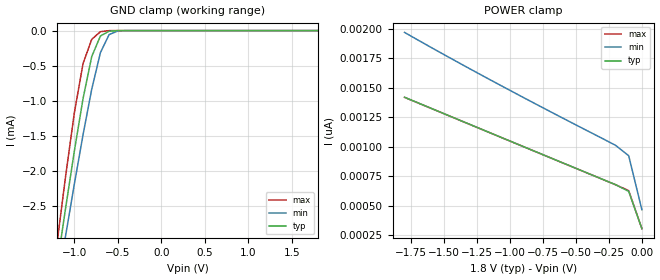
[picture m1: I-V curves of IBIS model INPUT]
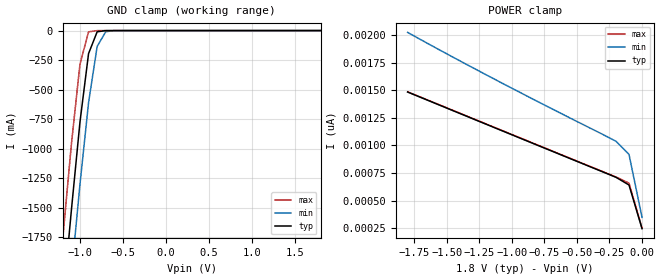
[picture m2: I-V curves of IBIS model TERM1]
|   PERICOM SEMICONDUCTOR CORP
|   IBIS Model of PI3CH360
|   Product Family: 3CH
|   TSSOP (L) Package
[IBIS Ver] 3.2
[Comment char] |_char
[File Name] pi3ch360_l_18v.ibs
[File Rev] 1.0
[Source] File originated at Pericom Semiconductor Corp.
[Date] 3/18/15
[Disclaimer] (C) Copyright PERICOM Semiconductor Corporation
   All rights reserved
  Pericom Semiconductor Corporation hereby grants the user of
  this IBIS model a non-exclusive, nontransferable license to
  use this IBIS model under the following terms.
  This IBIS model is provided on an "AS IS" basis and Pericom
  makes absolutely no warranty with respect to the information
  contained herein. PERICOM DISCLAIMS AND CUSTOMER WAIVES ALL
  WARRANTIES, EXPRESSED OR IMPLIED, INCLUDING WARRANTIES OF
  MERCHANTABILITY OR FITNESS FOR A PARTICULAR PURPOSE. The
  entire risk as to quality and performance is with the customer.
  Accordingly, in no event shall the company be liable for any
  damages, whether in contract or tort, including any lost
  profits or other incidental, consequential, exemplary, or
  punitive damages arising out of the use or application of the
  IBIS model provided in this package. Further, Pericom reserves
  the right to make changes without notice to any product herein
  to improve reliability, function, or design. Pericom does not
  convey any license under patent rights or any other intellectual
  property rights, including those of third parties.
  The user is granted this license only to use the IBIS model
  and is not granted rights to sell, load, rent, lease or license
  the IBIS model in whole or in part, or in modified form to anyone
  other than user. User may modify the IBIS model to suit its specific
  application but rights to derivative works and such modifications
  shall belong to Pericom.
  Pericom is not obligated to provide maintenance or support
  for the licensed IBIS model.
  Contact Pericom at ATTN: APPLICATION ENGINEERING / IBIS MODELS
  3545 North First Street, San Jose, CA 95134
[Component] PI3CH360
[Manufacturer] Pericom Semiconductor Corp.
[Package]
| variable   typ   min   max
R_pkg   0.05666ohm   0.05334ohm   0.05997ohm
L_pkg   2.99150nH   2.22200nH   3.76100nH
C_pkg   0.20800pF   0.16300pF   0.25300pF
[Pin]  signal_name   model_name   R_pin   L_pin   C_pin
1   S   INPUT   0.05997   3.76100nH   0.25300pF
2   NC   NC   0.05776   3.24800nH   0.22300pF
3   NC   NC   0.05555   2.73500nH   0.19300pF
4   YA   TERM2   0.05334   2.22200nH   0.16300pF
5   YB   TERM2   0.05334   2.22200nH   0.16300pF
6   YC   TERM2   0.05555   2.73500nH   0.19300pF
7   NC   NC   0.05776   3.24800nH   0.22300pF
8   GND   GND   0.05997   3.76100nH   0.25300pF
9   IC1   TERM1   0.05997   3.76100nH   0.25300pF
10   IB1   TERM1   0.05776   3.24800nH   0.22300pF
11   IA1   TERM1   0.05555   2.73500nH   0.19300pF
12   IC0   TERM1   0.05334   2.22200nH   0.16300pF
13   IB0   TERM1   0.05334   2.22200nH   0.16300pF
14   IA0   TERM1   0.05555   2.73500nH   0.19300pF
15   /EN   INPUT   0.05776   3.24800nH   0.22300pF
16   VCC   POWER   0.05997   3.76100nH   0.25300pF
[Series Switch Groups]
On 1 /
Off 2 /
[Series Pin Mapping]   pin_2   model_name  function_table_group
14   4   SWITCH1   1
13   5   SWITCH1   1
12   6   SWITCH1   1
11   4   SWITCH1   2
10   5   SWITCH1   2
9   6   SWITCH1   2
|   Model SWITCH1
[Model] SWITCH1
Model_type Series_switch
| variable   typ   min   max
C_comp   6.40pF   6.30pF   6.50pF
[Voltage Range]   1.800V   1.620V   1.980V
[GND Clamp Reference]   0.000V   0.000V   0.000V
[POWER Clamp Reference]   1.800V   1.620V   1.980V
[On]
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[OFF]
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| Models and submodels in the file (4): INPUT (Input), SWITCH1 (Series_switch), TERM1 (Terminator), TERM2 (Terminator)
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|   Model INPUT
[Model] INPUT
Model_type Input
Vinl = 0.600V
Vinh = 1.200V
| variable   typ   min   max
C_comp   1.800pF   1.700pF   1.900pF
[Voltage Range]   1.800V   1.620V   1.980V
[GND Clamp Reference]   0.000V   0.000V   0.000V
[POWER Clamp Reference]   1.800V   1.620V   1.980V
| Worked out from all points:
|   GND clamp passes 1 mA (typ) near -0.90 V on its own axis
[GND Clamp]
| Voltage   I(typ)   I(min)   I(max)
-1.8V     -8.577mA   -8.286mA   -9.176mA
-1.2V     -3.364mA   -3.668mA   -3.042mA
-1.1V     -2.528mA   -2.921mA   -2.075mA
-1V       -1.72mA    -2.189mA   -1.175mA
-900mV    -970.6uA   -1.485mA   -470.9uA
-800mV    -370.2uA   -835.9uA   -124.8uA
-700mV    -77.27uA   -313.6uA   -15.69uA
-600mV    -8.132uA   -56.97uA   -899.1nA
-500mV    -581.9nA   -5.514uA   -27.4nA
1.8V      304.9pA    998.4pA    16.08pA
[POWER Clamp]   |Note: Vtable = Vcc - Voutput
| Voltage   I(typ)   I(min)   I(max)
-1.8V     1.418nA    1.968nA    1.417nA
-1.1V     1.093nA    1.536nA    1.093nA
-200mV    677.5pA    1.011nA    677pA
-100mV    620.2pA    922.6pA    627.1pA
0V        304.9pA    464.9pA    304.7pA
|   Model TERM1
[Model] TERM1
Model_type Terminator
| variable   typ   min   max
C_comp   3.200pF   3.150pF   3.350pF
[Voltage Range]   1.800V   1.620V   1.980V
[GND Clamp Reference]   0.000V   0.000V   0.000V
[POWER Clamp Reference]   1.800V   1.620V   1.980V
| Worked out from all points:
|   GND clamp passes 1 mA (typ) near -0.71 V on its own axis
[GND Clamp]
| Voltage   I(typ)   I(min)   I(max)
-1.8V     -7.058A    -7.466A    -6.642A
-1.2V     -2.312A    -2.839A    -1.76A
-1.1V     -1.522A    -2.068A    -964.6mA
-1V       -774.2mA   -1.302A    -284.3mA
-900mV    -194.8mA   -609.8mA   -10.79mA
-800mV    -10.29mA   -134.3mA   -176uA
-700mV    -369.5uA   -9.267mA   -1.644uA
-500mV    -244.1nA   -27.85uA   -123.6pA
1.8V      244.8pA    1.023nA    53.58pA
[POWER Clamp]   |Note: Vtable = Vcc - Voutput
| Voltage   I(typ)   I(min)  I(max)
-1.8V     1.483nA    2.023nA    1.485nA
-1.1V     1.144nA    1.579nA    1.147nA
-200mV    710.2pA    1.037nA    713pA
-100mV    640.5pA    917.3pA    657.4pA
0V        244.8pA    347.1pA    248.7pA
